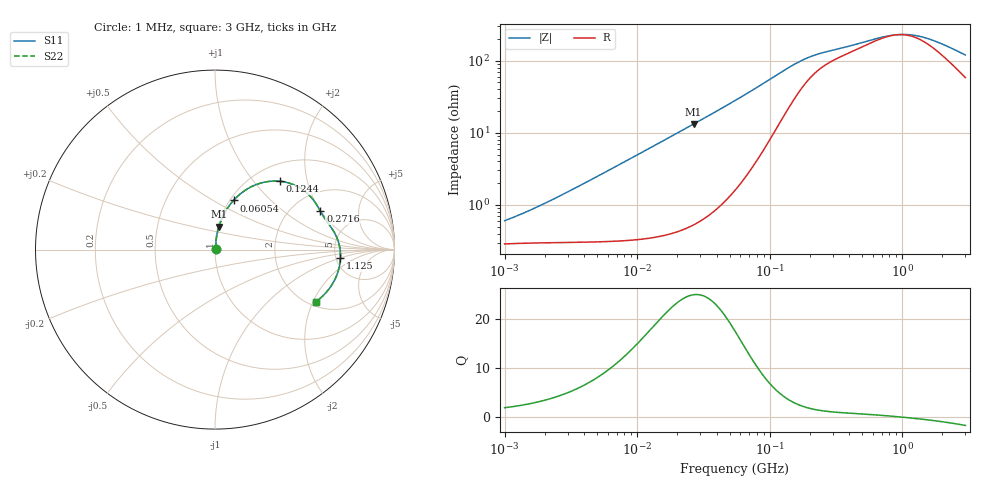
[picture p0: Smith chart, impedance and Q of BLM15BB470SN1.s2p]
! BLM15BB470SN1
# Hz S RI R 50
!Freq.(Hz) S11(Real) S11(Imag) S21(Real) S21(Imag) S12(Real) S12(Imag) S22(Real) S22(Imag)
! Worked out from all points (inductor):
!   401 points, 1 MHz to 3 GHz, reference 50 ohm
!   read as one part in series: L = 79.4 nH near 1.787 MHz
!   highest Q = 25.1 at 26.65 MHz (marker M1), where L = 78.8 nH
!   self-resonance near 921.6 MHz
!   S11 on the Smith chart (normalised r, x): 1 MHz: 1.01, +0.01; 60.54 MHz: 1.04, +0.62; 124.4 MHz: 1.31, +1.38; 271.6 MHz: 2.81, +1.98; 1.125 GHz: 5.49, -1.01; 3 GHz: 2.17, -2.10
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1000000  0.00289 0.00526  0.9971 -0.00526  0.9971 -0.00526  0.00289 0.00526
1751453  0.00303 0.00877  0.997 -0.00877  0.997 -0.00877  0.00303 0.00877
3823119  0.00337 0.0187  0.9966 -0.0187  0.9966 -0.0187  0.00337 0.0187
8017732  0.00471 0.0391  0.9953 -0.0391  0.9953 -0.0391  0.00471 0.0391
1.461624e7  0.00871 0.071  0.9913 -0.071  0.9913 -0.071  0.00871 0.071
2.664524e7  0.0221 0.1284  0.9779 -0.1284  0.9779 -0.1284  0.0221 0.1284
3.976269e7  0.0459 0.1885  0.9541 -0.1885  0.9541 -0.1885  0.0459 0.1885
5.477226e7  0.085 0.2519  0.915 -0.2519  0.915 -0.2519  0.085 0.2519
6.053752e7  0.1032 0.2739  0.8968 -0.2739  0.8968 -0.2739  0.1032 0.2739
8.507507e7  0.1971 0.3475  0.8029 -0.3475  0.8029 -0.3475  0.1971 0.3475
1.039275e8  0.2786 0.3764  0.7214 -0.3764  0.7214 -0.3764  0.2786 0.3764
1.244416e8  0.3632 0.3805  0.6368 -0.3805  0.6368 -0.3805  0.3632 0.3805
1.646891e8  0.484 0.3369  0.516 -0.3369  0.516 -0.3369  0.484 0.3369
2.094008e8  0.5495 0.2742  0.4505 -0.2742  0.4505 -0.2742  0.5495 0.2742
2.716345e8  0.5869 0.2147  0.4131 -0.2147  0.4131 -0.2147  0.5869 0.2147
5.473095e8  0.6599 0.1041  0.3401 -0.1041  0.3401 -0.1041  0.6599 0.1041
8.005644e8  0.6909 0.0311  0.3091 -0.0311  0.3091 -0.0311  0.6909 0.0311
9.585869e8  0.698 -0.00901  0.302 0.00901  0.302 0.00901  0.698 -0.00901
1.125055e9  0.699 -0.047  0.301 0.047  0.301 0.047  0.699 -0.047
1.430499e9  0.69 -0.1072  0.31 0.1072  0.31 0.1072  0.69 -0.1072
1.855641e9  0.6636 -0.1747  0.3364 0.1747  0.3364 0.1747  0.6636 -0.1747
3e9  0.5613 -0.2908  0.4387 0.2908  0.4387 0.2908  0.5613 -0.2908
